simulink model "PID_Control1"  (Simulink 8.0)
settings: Solver=ode3  StartTime=0.0  StopTime=inf  RelTol=1e-3
InitFcn:
  | dt=0.01;
  | %Kp=1.0; Kd=0; Ki=0;
undefined symbols (not defined in the file or in its folder): DiscIntNeverNeededParam
libraries: arduinolib x4, simulink x1

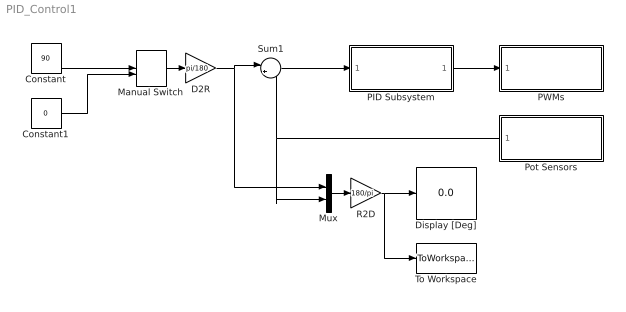
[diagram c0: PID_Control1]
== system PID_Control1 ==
  Constant : Constant  Value=90
  Constant1 : Constant  Value=0
  D2R : Gain  Gain=pi/180
  Display [Deg] : Display
  Manual Switch : ManualSwitch  CurrentSetting=0
  Mux : Mux  Inputs=2
  PID Subsystem : Subsystem  TreatAsAtomicUnit=on
  PWMs : Subsystem  TreatAsAtomicUnit=on
  Pot Sensors : Subsystem  TreatAsAtomicUnit=on
  R2D : Gain  Gain=180/pi
  Sum1 : Sum  Inputs=|+-
  To Workspace : ToWorkspace  VariableName=simout  SampleTime=-1  SaveFormat=Structure With Time
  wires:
  PID Subsystem/1(Out) -> PWMs/1(In1)
  Sum1/1 -> PID Subsystem/1(In)
  Pot Sensors/1(Out1) -> Mux/2, Sum1/2
  Manual Switch/1 -> D2R/1
  Constant/1 -> Manual Switch/1
  Constant1/1 -> Manual Switch/2
  D2R/1 -> Sum1/1, Mux/1
  Mux/1 -> R2D/1
  R2D/1 -> To Workspace/1, Display [Deg]/1

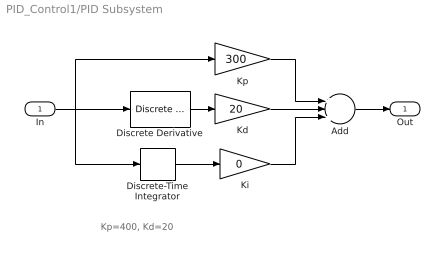
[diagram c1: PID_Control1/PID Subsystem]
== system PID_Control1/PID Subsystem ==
  note: Kp=400, Kd=20
  In : Inport
  Add : Sum  Inputs=+++
  Discrete Derivative : simulink/Discrete/Discrete Derivative  gainval=1.0  ICPrevScaledInput=0.0  InputProcessing=Inherited  OutMin=[]  OutMax=[]  OutDataType=fixdt(1, 16)  OutScaling=2^-10  DoSatur=off
  Discrete-Time Integrator : DiscreteIntegrator  SampleTime=dt  ICPrevOutput=DiscIntNeverNeededParam  ICPrevScaledInput=DiscIntNeverNeededParam
  Kd : Gain  Gain=20
  Ki : Gain  Gain=0
  Kp : Gain  Gain=300
  Out : Outport
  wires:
  Discrete-Time Integrator/1 -> Ki/1
  Kp/1 -> Add/1
  Kd/1 -> Add/2
  Ki/1 -> Add/3
  Discrete Derivative/1 -> Kd/1
  Add/1 -> Out/1
  In/1 -> Kp/1, Discrete Derivative/1, Discrete-Time Integrator/1

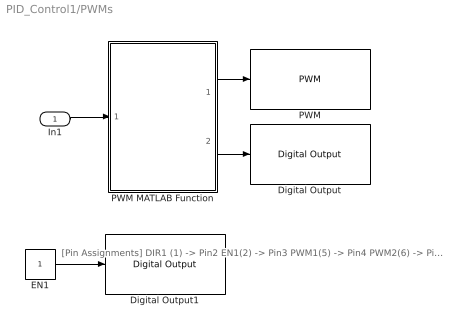
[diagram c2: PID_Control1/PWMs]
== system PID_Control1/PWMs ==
  note: [Pin Assignments] DIR1 (1) -> Pin2 EN1(2) -> Pin3 PWM1(5) -> Pin4 PWM2(6) -> Pin5 DIR2 (7) -> Pin6 EN2(8) -> Pin7
  In1 : Inport
  Digital Output : arduinolib/Digital Output  pinNumber=2
  Digital Output1 : arduinolib/Digital Output  pinNumber=3
  EN1 : Constant
  PWM : arduinolib/PWM  pinNumber=4
  PWM MATLAB Function : MATLAB Function  TreatAsAtomicUnit=on
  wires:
  EN1/1 -> Digital Output1/1
  PWM MATLAB Function/1(pwm) -> PWM/1
  PWM MATLAB Function/2(dir) -> Digital Output/1
  In1/1 -> PWM MATLAB Function/1(u)

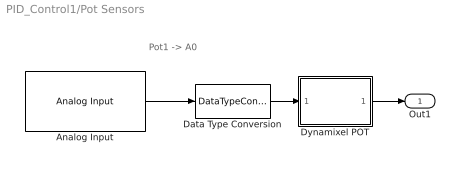
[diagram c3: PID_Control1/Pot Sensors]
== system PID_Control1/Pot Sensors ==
  note: Pot1 -> A0
  Analog Input : arduinolib/Analog Input  pinNumber=0  sampleTime=dt
  Data Type Conversion : DataTypeConversion  OutDataTypeStr=double
  Dynamixel POT : MATLAB Function  TreatAsAtomicUnit=on
  Out1 : Outport
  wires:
  Data Type Conversion/1 -> Dynamixel POT/1(u)
  Dynamixel POT/1(y) -> Out1/1
  Analog Input/1 -> Data Type Conversion/1

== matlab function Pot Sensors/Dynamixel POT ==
function y = fcn(u)
y=(pi/180)*(300/1024)*(u-204.8);

== matlab function PWMs/PWM
MATLAB Function ==
function [pwm, dir] = fcn(u)

if u>=0, dir=1;
else dir=0; end
pwm=abs(u);

% Saturation %
if pwm>=255, pwm=255; end
